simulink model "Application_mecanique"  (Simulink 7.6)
settings: Solver=ode15s  StartTime=0.0  StopTime=N  RelTol=1e-3
InitFcn:
  | N=2;
  | 
  | J=0.01;
  | fr=0.1;
  | k=10;
StopFcn:
  | close all
  | load pos_vit.mat
  | plotyy(x(1,:),x(2,:),x(1,:),x(4,:))
  | title('position et vitesse angulaires')
  | xlabel('temps')
  | grid
libraries: fl_lib x9, nesl_utility x6, AppliMechanical_lib x1

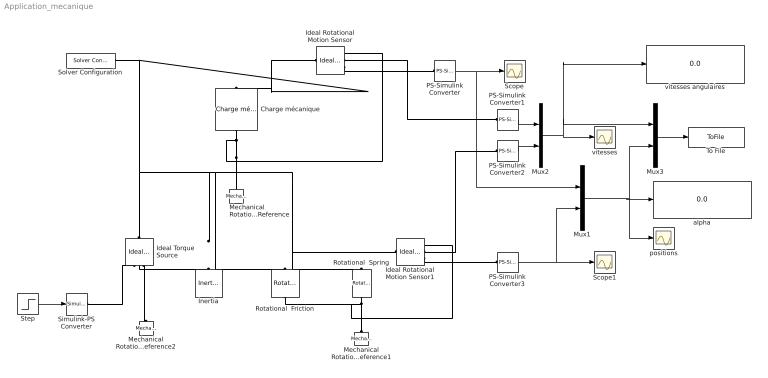
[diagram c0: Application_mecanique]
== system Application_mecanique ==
  Charge mécanique : AppliMechanical_lib/Charge mécanique  DialogController=NetworkEngine.DynNeDlgSource  SystemSampleTime=-1  k=k N*m/rad  J=J kg*m^2  fr=fr N*m/(rad/s)  alpha_Log=off  t_Log=off  w_Log=off  LocalVarNames=|alpha|t|w  LocalVarDescs=|alpha|t|w  LocalVarLogging=[0 0 0]
  Ideal Rotational Motion Sensor : fl_lib/Mechanical/Mechanical Sensors/Ideal Rotational Motion Sensor  DialogController=NetworkEngine.DynNeDlgSource  SystemSampleTime=-1  offset=0 rad  w_Log=off  t_Log=off  phi_Log=off  LocalVarNames=|w|t|phi  LocalVarDescs=|w|t|phi  LocalVarLogging=[0 0 0]
  Ideal Rotational Motion Sensor1 : fl_lib/Mechanical/Mechanical Sensors/Ideal Rotational Motion Sensor  DialogController=NetworkEngine.DynNeDlgSource  SystemSampleTime=-1  offset=0 rad  w_Log=off  t_Log=off  phi_Log=off  LocalVarNames=|w|t|phi  LocalVarDescs=|w|t|phi  LocalVarLogging=[0 0 0]
  Ideal Torque  Source : fl_lib/Mechanical/Mechanical Sources/Ideal Torque Source  DialogController=NetworkEngine.DynNeDlgSource  SystemSampleTime=-1  w_Log=off  t_Log=off  LocalVarNames=|w|t  LocalVarDescs=|w|t  LocalVarLogging=[0 0]
  Inertia : fl_lib/Mechanical/Rotational Elements/Inertia  DialogController=NetworkEngine.DynNeDlgSource  SystemSampleTime=-1  inertia=J kg*m^2  initial_velocity=0 rad/s  t_Log=off  LocalVarNames=|t  LocalVarDescs=|t  LocalVarLogging=0
  Mechanical Rotational Reference : fl_lib/Mechanical/Rotational Elements/Mechanical Rotational Reference  DialogController=NetworkEngine.DynNeDlgSource  SystemSampleTime=-1  t_Log=off  LocalVarNames=|t  LocalVarDescs=|t  LocalVarLogging=0
  Mechanical Rotational Reference1 : fl_lib/Mechanical/Rotational Elements/Mechanical Rotational Reference  DialogController=NetworkEngine.DynNeDlgSource  SystemSampleTime=-1  t_Log=off  LocalVarNames=|t  LocalVarDescs=|t  LocalVarLogging=0
  Mechanical Rotational Reference2 : fl_lib/Mechanical/Rotational Elements/Mechanical Rotational Reference  DialogController=NetworkEngine.DynNeDlgSource  SystemSampleTime=-1  t_Log=off  LocalVarNames=|t  LocalVarDescs=|t  LocalVarLogging=0
  Mux1 : Mux  Inputs=2
  Mux2 : Mux  Inputs=2
  Mux3 : Mux  Inputs=2
  PS-Simulink Converter{,1..3} (4 alike) : nesl_utility/PS-Simulink Converter  DialogController=NetworkEngine.DynNeUtilDlgSource  SystemSampleTime=-1  PhysicalDomain=network_engine_domain  LeftPortType=input  RightPortType=output  SubClassName=ps_output  Unit=1  AffineConversion=off
  Rotational  Friction : fl_lib/Mechanical/Rotational Elements/Rotational Friction  DialogController=NetworkEngine.DynNeDlgSource  SystemSampleTime=-1  brkwy_trq=1e-9 N*m  Col_trq=1e-9 N*m  visc_coef=fr N*m/(rad/s)  trans_coef=1e-9 s/rad  vel_thr=1e-9 rad/s  t_Log=off  w_Log=off  LocalVarNames=|t|w  LocalVarDescs=|t|w  LocalVarLogging=[0 0]
  Rotational  Spring : fl_lib/Mechanical/Rotational Elements/Rotational Spring  DialogController=NetworkEngine.DynNeDlgSource  SystemSampleTime=-1  spr_rate=k N*m/rad  init_def=0 rad  t_Log=off  w_Log=off  phi_Log=off  LocalVarNames=|t|w|phi  LocalVarDescs=|t|w|phi  LocalVarLogging=[0 0 0]
  Scope : Scope
  Scope1 : Scope
  Simulink-PS Converter : nesl_utility/Simulink-PS Converter  DialogController=NetworkEngine.DynNeUtilDlgSource  SystemSampleTime=-1  PhysicalDomain=network_engine_domain  LeftPortType=input  RightPortType=output  SubClassName=ps_input  Unit=1  AffineConversion=off  InputFilterTimeConstant=.001  UdotUserProvided=0
  Solver Configuration : nesl_utility/Solver Configuration  DialogController=NetworkEngine.DynNeUtilDlgSource  SystemSampleTime=-1  PhysicalDomain=network_engine_domain  LeftPortType=input  RightPortType=generic  SubClassName=solver  Accelerate=off  Profile=off  ResidualTolerance=1e-9  MaxNonlinIter=3  MaxModeIter=2  DoFixedCost=off  UseLocalSampling=off  DoDC=off  LinearAlgebra=Sparse  LocalSolverSampleTime=.001  LocalSolverChoice=NE_BACKWARD_EULER_ADVANCER  UseLocalSolver=off
  Step : Step  Time=0.02  After=10  SampleTime=0
  To File : ToFile  Filename=pos_vit  MatrixName=x
  alpha : Display
  positions : Scope
  vitesses : Scope
  vitesses angulaires : Display
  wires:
  Step/1 -> Simulink-PS Converter/1
  PS-Simulink Converter3/1 -> Scope1/1, Mux1/2
  PS-Simulink Converter/1 -> Scope/1, Mux1/1
  Mux1/1 -> alpha/1, Mux3/2, positions/1
  PS-Simulink Converter1/1 -> Mux2/1
  PS-Simulink Converter2/1 -> Mux2/2
  Mux2/1 -> vitesses/1, vitesses angulaires/1, Mux3/1
  Mux3/1 -> To File/1
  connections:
  Charge mécanique/RConn1 -- Mechanical Rotational Reference/LConn1 -- Ideal Rotational Motion Sensor/RConn1
  Simulink-PS Converter/RConn1 -- Ideal Torque  Source/RConn1
  Rotational  Friction/RConn1 -- Rotational  Spring/RConn1 -- Mechanical Rotational Reference1/LConn1 -- Ideal Rotational Motion Sensor1/RConn1
  Ideal Rotational Motion Sensor1/RConn3 -- PS-Simulink Converter3/LConn1
  Ideal Rotational Motion Sensor/RConn3 -- PS-Simulink Converter/LConn1
  Ideal Rotational Motion Sensor/RConn2 -- PS-Simulink Converter1/LConn1
  PS-Simulink Converter2/LConn1 -- Ideal Rotational Motion Sensor1/RConn2
  Inertia/LConn1 -- Rotational  Friction/LConn1 -- Rotational  Spring/LConn1 -- Ideal Rotational Motion Sensor1/LConn1 -- Ideal Rotational Motion Sensor/LConn1 -- Charge mécanique/LConn1 -- Solver Configuration/RConn1 -- Ideal Torque  Source/LConn1
  Ideal Torque  Source/RConn2 -- Mechanical Rotational Reference2/LConn1
